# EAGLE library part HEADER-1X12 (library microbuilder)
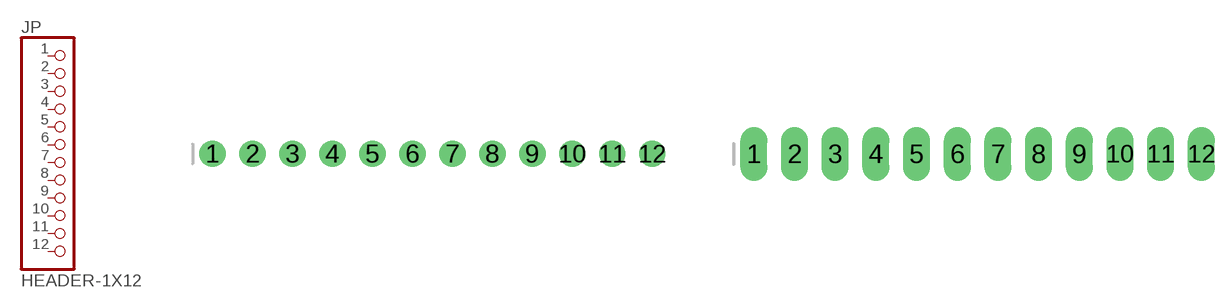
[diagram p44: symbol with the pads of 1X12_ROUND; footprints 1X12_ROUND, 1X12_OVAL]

Designator prefix JP

## HEADER-1X12  [1X12_ROUND]
1  1  pas
2  2  pas
3  3  pas
4  4  pas
5  5  pas
6  6  pas
7  7  pas
8  8  pas
9  9  pas
10  10  pas
11  11  pas
12  12  pas

## HEADER-1X12OVAL  [1X12_OVAL]
Pads as for 1X12_ROUND

## HEADER-1X1280MIL  [1X12_ROUND_80MIL]
Pads as for 1X12_ROUND

## HEADER-1X1276MIL  [1X12_ROUND_76MIL]
Pads as for 1X12_ROUND

## Footprint 1X12_ROUND (pad centres in mm)
drill 1 pad 1.676: 1 -13.97,0; 2 -11.43,0; 3 -8.89,0; 4 -6.35,0; 5 -3.81,0; 6 -1.27,0; 7 1.27,0; 8 3.81,0; 9 6.35,0; 10 8.89,0; 11 11.43,0; 12 13.97,0

## Footprint 1X12_OVAL (pad centres in mm)
drill 1 pad 1.676 long: 1 -13.97,0; 2 -11.43,0; 3 -8.89,0; 4 -6.35,0; 5 -3.81,0; 6 -1.27,0; 7 1.27,0; 8 3.81,0; 9 6.35,0; 10 8.89,0; 11 11.43,0; 12 13.97,0

## Footprint 1X12_ROUND_80MIL (pad centres in mm)
drill 1 pad 2.032: 1 -13.97,0; 2 -11.43,0; 3 -8.89,0; 4 -6.35,0; 5 -3.81,0; 6 -1.27,0; 7 1.27,0; 8 3.81,0; 9 6.35,0; 10 8.89,0; 11 11.43,0; 12 13.97,0

## Footprint 1X12_ROUND_76MIL (pad centres in mm)
drill 1 pad 1.93: 1 -13.97,0; 2 -11.43,0; 3 -8.89,0; 4 -6.35,0; 5 -3.81,0; 6 -1.27,0; 7 1.27,0; 8 3.81,0; 9 6.35,0; 10 8.89,0; 11 11.43,0; 12 13.97,0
